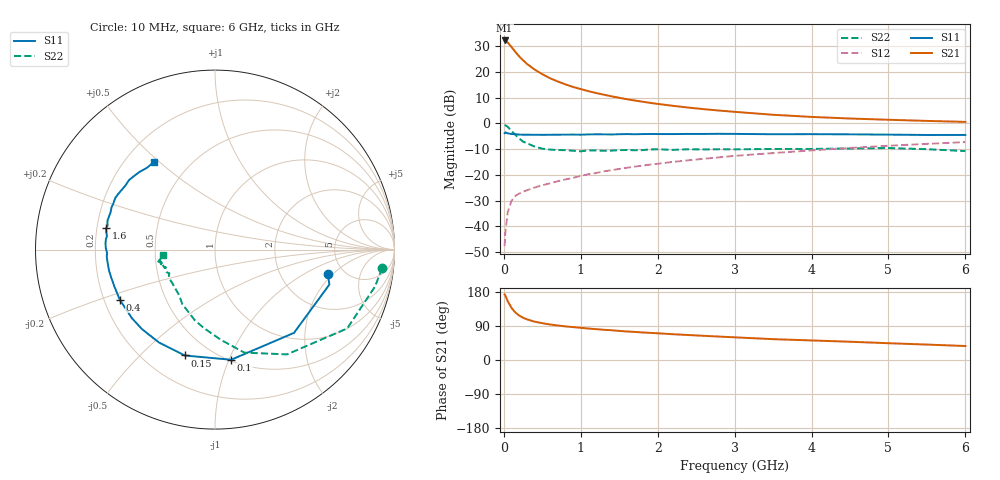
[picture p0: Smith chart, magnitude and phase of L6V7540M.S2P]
!  INFINEON TECHNOLOGIES Small Signal Semiconductors
! BFR380L3 , Si-NPN RF-Transistor in TSLP-3-1
!  Vce=0.75 V,  Ic=40 mA
! Common Emitter S-Parameters:  07. March 2005
#  GHz  S  MA  R  50
! f  S11  S21  S12  S22
! GHz  Mag  Ang  Mag  Ang  Mag  Ang  Mag  Ang
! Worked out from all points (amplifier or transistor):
!   36 points, 10 MHz to 6 GHz, reference 50 ohm
!   highest |S21| = 32.2 dB at 10 MHz (marker M1)
!   |S21| within 3 dB of that: start of sweep to 111.9 MHz
!   unconditionally stable (mu >= 1): 1.289 GHz to end of sweep
!   at 250 MHz: K = 0.49, MSG = 25.5 dB, |S12| = -26.6 dB
!   at 1.4 GHz: K = 1.02, MAG = 13.6 dB, |S12| = -18.2 dB
!   at 6 GHz: K = 1.00, MAG = 3.8 dB, |S12| = -7.3 dB
!   S11 on the Smith chart (normalised r, x): 10 MHz: 3.74, -1.77; 100 MHz: 0.51, -1.02; 150 MHz: 0.36, -0.69; 400 MHz: 0.26, -0.23; 1.6 GHz: 0.24, +0.09; 6 GHz: 0.32, +0.48
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0.01  0.6444 -12.4  40.76 173.1  0.0041 79.4  0.9368 -6.3
0.02  0.6663 -17.0  40.43 170.0  0.0077 82.9  0.9154 -12.9
0.05  0.6395 -46.5  37.27 155.5  0.0186 70.7  0.8575 -30.8
0.1  0.6202 -81.7  30.41 137.4  0.0313 58.2  0.7084 -55.5
0.15  0.6134 -105.9  24.4 125.2  0.0389 51.0  0.5969 -74.1
0.2  0.6045 -121.0  19.95 117.2  0.0432 48.5  0.5055 -86.0
0.25  0.6015 -132.6  16.78 111.6  0.0469 46.8  0.4415 -98.1
0.3  0.6003 -140.5  14.32 107.3  0.05 47.8  0.4081 -106.2
0.4  0.5994 -152.3  11.08 101.1  0.0565 48.2  0.3542 -120.9
0.5  0.5971 -159.7  9.006 97.1  0.0625 50.7  0.3211 -129.1
0.6  0.5989 -165.0  7.522 93.7  0.0681 52.6  0.3092 -136.0
0.7  0.6019 -168.9  6.51 91.1  0.075 55.1  0.3023 -142.3
0.9  0.6045 -176.3  5.089 86.8  0.0871 58.0  0.2933 -151.2
1.1  0.6085 179.2  4.213 83.0  0.1025 60.2  0.2967 -154.7
1.3  0.6104 174.3  3.598 79.7  0.1167 61.1  0.292 -160.7
1.6  0.6181 168.8  2.941 75.3  0.1369 62.1  0.3034 -164.3
2.2  0.6177 160.4  2.187 68.0  0.178 62.9  0.3049 -165.7
2.8  0.6254 152.6  1.771 61.8  0.2183 62.8  0.3137 -169.1
3.5  0.6136 144.4  1.466 55.0  0.2642 60.5  0.3174 -168.4
4.5  0.6103 138.1  1.24 48.2  0.3324 58.1  0.3245 -167.9
5.5  0.5932 129.9  1.114 40.7  0.3988 53.5  0.314 -169.4
6  0.5943 124.7  1.066 36.9  0.4319 51.1  0.2888 -174.2
